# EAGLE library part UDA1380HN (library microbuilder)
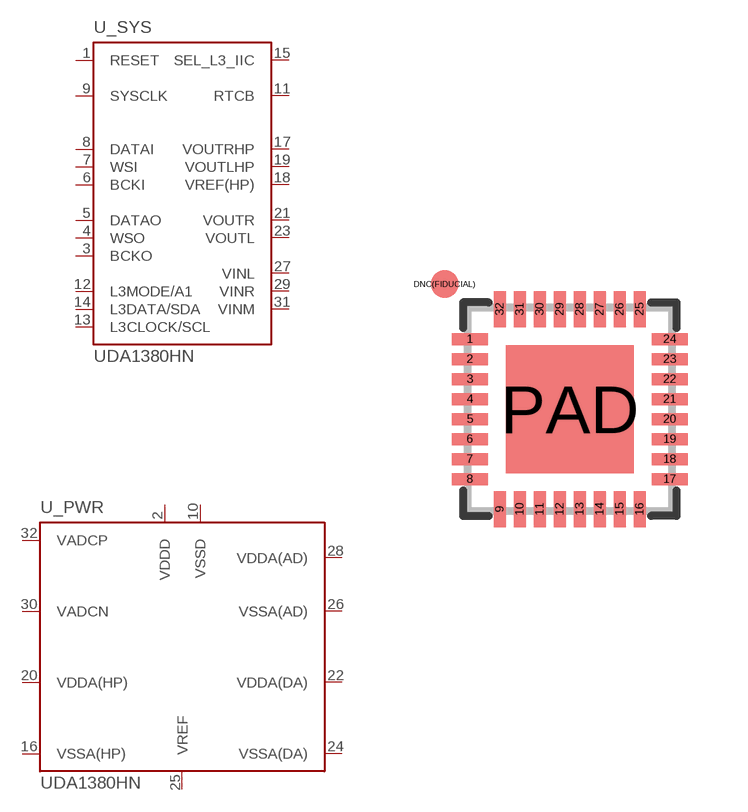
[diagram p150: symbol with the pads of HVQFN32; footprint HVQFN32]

Designator prefix U; gates _PWR=UDA1380_POWER _SYS=UDA1380

## UDA1380HN  [HVQFN32]
1  _SYS:RESET  in
2  _PWR:VDDD  pwr
3  _SYS:BCKO
4  _SYS:WSO
5  _SYS:DATAO  out
6  _SYS:BCKI  in
7  _SYS:WSI  in
8  _SYS:DATAI  in
9  _SYS:SYSCLK  in
10  _PWR:VSSD  pwr
11  _SYS:RTCB  in
12  _SYS:L3MODE/A1  in
13  _SYS:L3CLOCK/SCL  in
14  _SYS:L3DATA/SDA
15  _SYS:SEL_L3_IIC  in
16  _PWR:VSSA(HP)  pwr
17  _SYS:VOUTRHP  out
18  _SYS:VREF(HP)
19  _SYS:VOUTLHP  out
20  _PWR:VDDA(HP)  pwr
21  _SYS:VOUTR  out
22  _PWR:VDDA(DA)  pwr
23  _SYS:VOUTL  out
24  _PWR:VSSA(DA)  pwr
25  _PWR:VREF  pwr
26  _PWR:VSSA(AD)  pwr
27  _SYS:VINL  in
28  _PWR:VDDA(AD)  pwr
29  _SYS:VINR  in
30  _PWR:VADCN  pwr
31  _SYS:VINM  in
32  _PWR:VADCP  pwr

## Footprint HVQFN32 (pad centres in mm)
HVQFN32 SOT617-1 JEDEC MO-220
smd 0.9 x 0.3: 1 -2.5,1.75; 2 -2.5,1.25; 3 -2.5,0.75; 4 -2.5,0.25; 5 -2.5,-0.25; 6 -2.5,-0.75; 7 -2.5,-1.25; 8 -2.5,-1.75; 17 2.5,-1.75; 18 2.5,-1.25; 19 2.5,-0.75; 20 2.5,-0.25; 21 2.5,0.25; 22 2.5,0.75; 23 2.5,1.25; 24 2.5,1.75
smd 0.3 x 0.9: 9 -1.75,-2.5; 10 -1.25,-2.5; 11 -0.75,-2.5; 12 -0.25,-2.5; 13 0.25,-2.5; 14 0.75,-2.5; 15 1.25,-2.5; 16 1.75,-2.5; 25 1.75,2.5; 26 1.25,2.5; 27 0.75,2.5; 28 0.25,2.5; 29 -0.25,2.5; 30 -0.75,2.5; 31 -1.25,2.5; 32 -1.75,2.5
smd 0.7 x 0.7: DNC(FIDUCIAL) -3.127,3.127
smd 3.2 x 3.2: PAD 0,0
